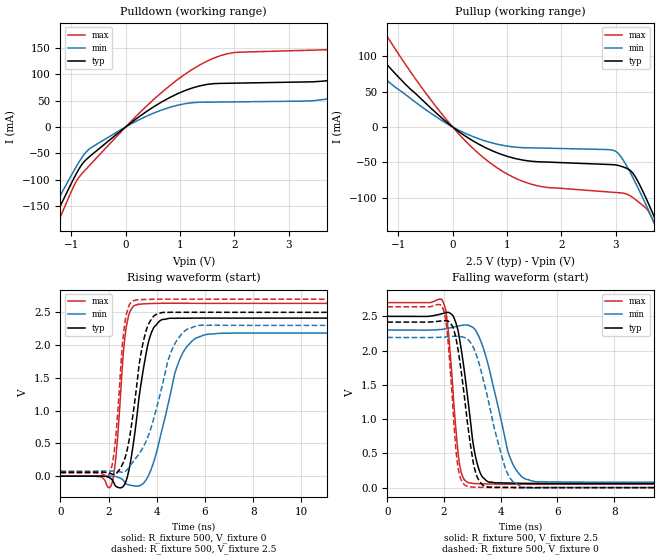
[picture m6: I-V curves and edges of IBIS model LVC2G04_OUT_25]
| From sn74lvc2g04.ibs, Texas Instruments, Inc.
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[Model]   LVC2G04_OUT_25
Model_type  Output
Vref =   0
Rref =   500
Cref =   30p
Vmeas =   1.25
| variable   typ   min   max
C_comp   9.70pF   6.16pF   13.61pF
| C_pullup   9.66pF   6.16pF   11.44pF
| C_pulldown   9.73pF   6.26pF   13.61pF
[Temperature Range]   40   100   -40
| Ambient temperature   25   85   -40
[Voltage range]   2.5   2.3   2.7
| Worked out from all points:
|   slope of the pulldown table from 0 to 0.375 V, typ, clamps not added: 13.1 ohm
|   slope of the pullup table from 0 to 0.375 V, typ, clamps not added: 19 ohm
|   rising waveform, R_fixture 500, V_fixture 0: 20-80 % time 565ps typ, 877ps min, 316ps max; typ from 0 V to 2.41 V
|   falling waveform, R_fixture 500, V_fixture 2.5: 20-80 % time 458ps typ, 741ps min, 303ps max; typ from 2.5 V to 0.06 V
|   rising waveform, R_fixture 500, V_fixture 2.5: 20-80 % time 568ps typ, 1.01ns min, 327ps max; typ from 0.06 V to 2.5 V
|   falling waveform, R_fixture 500, V_fixture 0: 20-80 % time 461ps typ, 776ps min, 279ps max; typ from 2.42 V to 0 V
[Pulldown]
| LVC2G04_OUT_25
|   Voltage   I(typ)   I(min)   I(max)
-5.5V     -1.065A    -962.2mA   -1.199A
-1.53V    -221.1mA   -193.8mA   -251.2mA
-1.17V    -142.7mA   -123.7mA   -162.8mA
-670mV    -56.67mA   -41.91mA   -73.36mA
520mV     38.43mA    26.46mA    52.49mA
1.485V    80.34mA    46.87mA    124mA
3.84V     90.07mA    55.63mA    147.9mA
5.34V     157.5mA    105.9mA    231.4mA
5.91V     188.7mA    52.63mA    282.8mA
6.525V    93.57mA    53.14mA    298.9mA
7.56V     94.12mA    54.12mA    160.7mA
11V       99.65mA    57.57mA    168.9mA
[Pullup]
| LVC2G04_OUT_25
|   Voltage   I(typ)   I(min)   I(max)
-5.5V     533.4mA    418.6mA    746.4mA
-2.34V    192.7mA    147.4mA    275.6mA
-1.735V   134.9mA    102mA      194.6mA
-1.32V    97.81mA    73.23mA    142.1mA
-135mV    8.418mA    6.055mA    12.49mA
750mV     -34.38mA   -23.05mA   -54.11mA
1.57V     -49.22mA   -29.81mA   -83.34mA
2.995V    -53.63mA   -34.3mA    -92.61mA
3.315V    -65.3mA    -71.46mA   -99.87mA
3.565V    -101.9mA   -111.4mA   -115.4mA
3.75V     -134.3mA   -142.6mA   -143.5mA
11V       -1.614A    -1.516A    -1.761A
[Ramp]
| LVC2G04_OUT_25
| variable   typ   min   max
dV/dt_r   1.55/6.14E-10   1.40/1.02E-09   1.69/3.42E-10
dV/dt_f   1.50/4.87E-10   1.38/7.93E-10   1.62/3.22E-10
R_load = 500
[Rising Waveform]
| LVC2G04_OUT_25
R_fixture =   500
C_fixture =   0
L_fixture =   0
V_fixture =   0
V_fixture_min = 0
V_fixture_max = 0
|   Time   V(typ)   V(min)   V(max)
0s        123.6pV    5.747nV    2.756nV
2.1ns     -38.22mV   344.9uV    -146.5mV
2.31ns    -156.7mV   -8.208mV   325.8mV
2.72ns    -76.89mV   -116.4mV   2.245V
3.21ns    1.03V      -150.2mV   2.621V
3.615ns   1.986V     -17.76mV   2.632V
3.9ns     2.279V     251.7mV    2.636V
4.925ns   2.41V      1.756V     2.638V
5.97ns    2.412V     2.155V     2.637V
24.99ns   2.411V     2.183V     2.637V
[Falling Waveform]
| LVC2G04_OUT_25
R_fixture =   500
C_fixture =   0
L_fixture =   0
V_fixture =   2.5
V_fixture_min = 2.3
V_fixture_max = 2.7
|   Time   V(typ)   V(min)   V(max)
0s        2.5V       2.3V       2.7V
1.965ns   2.543V     2.311V     2.713V
2.145ns   2.56V      2.326V     2.308V
2.535ns   2.201V     2.361V     377mV
2.885ns   1.142V     2.366V     67.91mV
3.1ns     476.1mV    2.301V     58.49mV
3.36ns    153.3mV    2.068V     55.15mV
4.315ns   66.81mV    455.3mV    49.14mV
5.135ns   61.25mV    93.95mV    48.93mV
24.99ns   60.11mV    77.11mV    49.35mV
[Rising Waveform]
| LVC2G04_OUT_25
R_fixture =   500
C_fixture =   0
L_fixture =   0
V_fixture =   2.5
V_fixture_min = 2.3
V_fixture_max = 2.7
|   Time   V(typ)   V(min)   V(max)
0s        60.06mV    77.04mV    49.31mV
2.055ns   43.44mV    78.13mV    58.51mV
2.28ns    27.16mV    75.08mV    539.4mV
2.67ns    267.7mV    68.61mV    2.327V
3.055ns   1.056V     240.1mV    2.682V
3.4ns     1.983V     419.3mV    2.694V
3.79ns    2.403V     773.7mV    2.699V
4.665ns   2.501V     1.958V     2.701V
5.655ns   2.501V     2.293V     2.7V
24.99ns   2.5V       2.3V       2.7V
[Falling Waveform]
| LVC2G04_OUT_25
R_fixture =   500
C_fixture =   0
L_fixture =   0
V_fixture =   0
V_fixture_min = 0
V_fixture_max = 0
|   Time   V(typ)   V(min)   V(max)
0s        2.416V     2.191V     2.64V
1.93ns    2.434V     2.196V     2.648V
2.12ns    2.434V     2.202V     2.239V
2.485ns   2.038V     2.208V     321.1mV
2.87ns    811.2mV    2.151V     14.06mV
3.085ns   267.7mV    2V         6.127mV
3.34ns    46.56mV    1.647V     3.737mV
4.16ns    4.126mV    282.8mV    -69.34uV
4.805ns   1.143mV    3.893mV    -383.6uV
24.99ns   41.37uV    58.09uV    34.34uV
